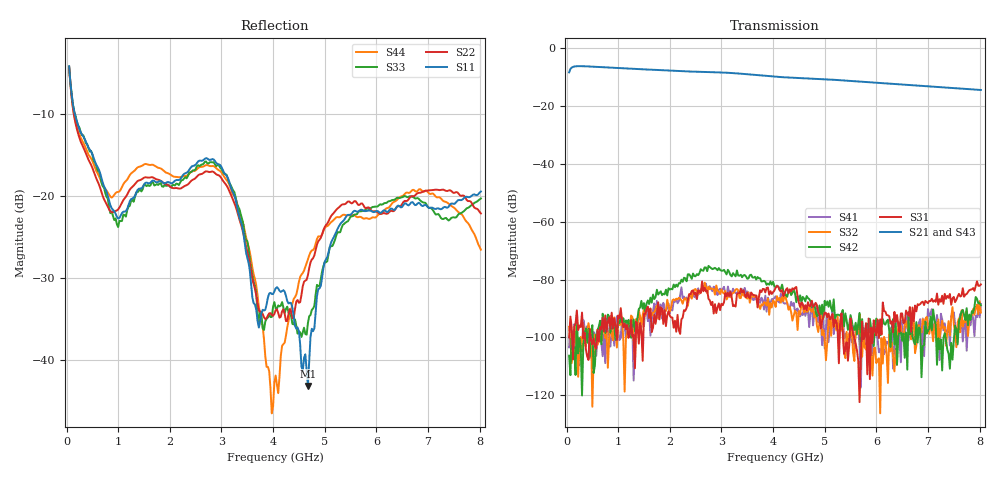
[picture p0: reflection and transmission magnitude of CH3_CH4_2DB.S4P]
!Agilent Technologies,E5071C,MY46316741,A.11.02
!Date: Thu May 28 15:03:59 2026
!Data & Calibration Information:
!1:CH3 INPUT 2:CH3 OUTPUT 3:CH4 INPUT 4:CH4 OUTPUT
!Freq	S11:SOLT4(ON)	S12:SOLT4(ON)	S13:SOLT4(ON)	S14:SOLT4(ON)
!	S21:SOLT4(ON)	S22:SOLT4(ON)	S23:SOLT4(ON)	S24:SOLT4(ON)
!	S31:SOLT4(ON)	S32:SOLT4(ON)	S33:SOLT4(ON)	S34:SOLT4(ON)
!	S41:SOLT4(ON)	S42:SOLT4(ON)	S43:SOLT4(ON)	S44:SOLT4(ON)
!PortZ  Port1:50+j0  Port2:50+j0  Port3:50+j0  Port4:50+j0
!Above PortZ is port z conversion or system Z0 setting when saving the data.
!When reading, reference impedance value at option line is always used.
# Hz S dB R 50
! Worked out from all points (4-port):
!   320 points, 50 MHz to 8.025 GHz, reference 50 ohm
!   strongest paths, dB at 50 MHz, 2.05 GHz, 4.05 GHz, 6.05 GHz, 8.025 GHz:
!     S21: -8.3, -7.7, -9.8, -12.0, -14.4
!     S43: -8.3, -7.8, -9.9, -12.1, -14.6
!     S31: -100.1, -93.2, -82.8, -100.3, -81.7
!     S42: -106.3, -83.4, -82.7, -94.2, -88.9
!     S32: -96.4, -87.2, -89.5, -107.3, -91.4
!     S41: -103.5, -90.7, -85.8, -105.2, -88.4
!   lowest |S11| = -43.2 dB at 4.675 GHz (marker M1), VSWR 1.01, Z = 49.4 - j0.381 ohm
!   |S11| at or under -10 dB: 159.6 MHz to end of sweep
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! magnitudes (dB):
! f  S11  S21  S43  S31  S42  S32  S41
! 50 MHz  -4.2  -8.3  -8.3  -100.1  -106.3  -96.4  -103.5
! 1 GHz  -22.8  -6.9  -6.9  -92.4  -94.9  -95.8  -97.4
! 3.125 GHz  -17.8  -8.5  -8.5  -84.6  -76.6  -86.0  -82.4
! 3.975 GHz  -32.0  -9.7  -9.8  -85.0  -81.8  -89.7  -86.8
! 4.675 GHz  -43.2  -10.4  -10.5  -87.8  -86.4  -91.0  -90.7
! 5.425 GHz  -22.5  -11.2  -11.2  -101.7  -94.1  -98.1  -100.9
! 8.025 GHz  -19.5  -14.4  -14.6  -81.7  -88.9  -91.4  -88.4
